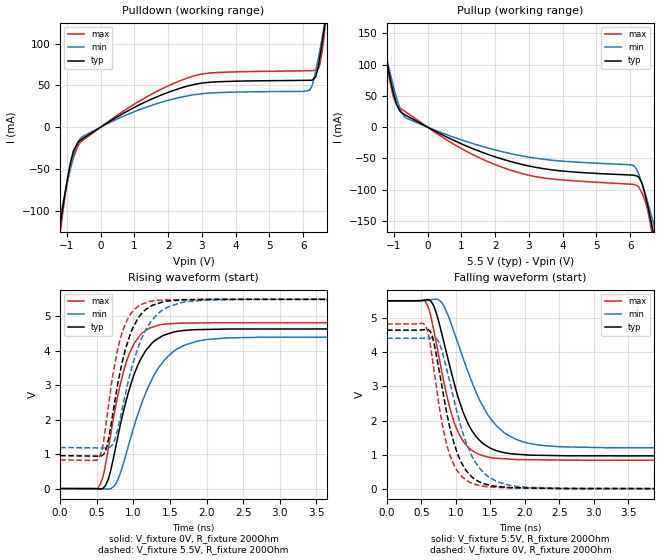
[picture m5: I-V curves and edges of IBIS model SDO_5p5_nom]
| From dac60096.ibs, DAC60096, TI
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|   Model
[Model]   SDO_5p5_nom
Model_type   Output
Polarity   Non-Inverting
Vmeas = 2.75
Vref = 0
Cref = 1pF
Rref = 100000
|   typ   min   max
C_comp   13.124pF   12.937pF   13.913pF
[Voltage Range]   5.5   5.499   5.501
[Temperature Range]   27   105   -40
[Pullup Reference]   5.5   5.499   5.501
[Pulldown Reference]   0   0   0
[Power Clamp Reference]   5.5   5.499   5.501
[GND Clamp Reference]   0   0   0
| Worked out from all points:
|   slope of the pulldown table from 0 to 0.825 V, typ, clamps not added: 41.5 ohm
|   slope of the pullup table from 0 to 0.825 V, typ, clamps not added: 36.9 ohm
|   falling waveform, V_fixture 5.5V, R_fixture 200Ohm: 20-80 % time 400ps typ, 541ps min, 325ps max; typ from 5.5 V to 0.955 V
|   rising waveform, V_fixture 0V, R_fixture 200Ohm: 20-80 % time 357ps typ, 464ps min, 292ps max; typ from 0 V to 4.64 V
|   rising waveform, V_fixture 5.5V, R_fixture 200Ohm: 20-80 % time 282ps typ, 354ps min, 233ps max; typ from 0.955 V to 5.5 V
|   falling waveform, V_fixture 0V, R_fixture 200Ohm: 20-80 % time 309ps typ, 390ps min, 263ps max; typ from 4.64 V to 0 V
[Pulldown]
|   Voltage   I(typ)   I(min)   I(max)
-5.5V     -1.396A    -1.141A    -1.674A
-1.359V   -160.1mA   -141.1mA   -181mA
-1.144V   -102mA     -96.41mA   -109.2mA
-995.5mV  -64.53mA   -67.3mA    -67.28mA
-814mV    -29.52mA   -35.59mA   -37.78mA
-566.5mV  -14.69mA   -12.25mA   -16.91mA
2.733V    50.8mA     38.61mA    61.04mA
6.182V    56.1mA     44.1mA     67.53mA
6.364V    59.98mA    65.71mA    68.08mA
6.479V    80.55mA    89.03mA    72.98mA
6.677V    133.5mA    133.4mA    129.2mA
11V       1.487A     1.216A     1.844A
[Pullup]
|   Voltage   I(typ)   I(min)   I(max)
-5.5V     1.434A     1.169A     1.793A
-1.837V   293.1mA    259.1mA    340.4mA
-1.375V   153.7mA    148mA      162.9mA
-1.095V   74.62mA    83.43mA    67.54mA
-814mV    25.31mA    29.59mA    30.55mA
-38.5mV   1.133mA    858.2uA    1.477mA
2.321V    -52.9mA    -40.63mA   -66.35mA
6.099V    -76.87mA   -61.46mA   -91.65mA
6.347V    -89.44mA   -88.99mA   -104.8mA
6.644V    -157.3mA   -144.3mA   -168.5mA
6.726V    -179.2mA   -161.1mA   -195.4mA
11V       -1.454A    -1.191A    -1.738A
[Ramp]
R_load = 200
|   typ   min   max
dV/dt_r   2.78525/3.57276e-10   2.64196/4.63284e-10   2.89374/2.91791e-10
dV/dt_f   2.72682/4e-10   2.58421/5.38847e-10   2.80226/3.25162e-10
[Falling Waveform]
V_fixture = 5.5V
V_fixture_min = 5.499V
V_fixture_max = 5.501V
R_fixture = 200Ohm
C_fixture = 0F
|   Time   V(typ)   V(min)   V(max)
0s        5.5V       5.499V     5.501V
539.6ps   5.518V     5.499V     5.5V
650.8ps   5.447V     5.53V      4.907V
810.9ps   4.406V     5.394V     3.264V
997ps     2.928V     4.444V     1.83V
1.198ns   1.826V     3.306V     1.188V
1.445ns   1.263V     2.229V     945.6mV
1.867ns   1.023V     1.459V     865.8mV
2.505ns   978.5mV    1.238V     848.7mV
10ns      955.3mV    1.192V     830.6mV
[Rising Waveform]
V_fixture = 0V
V_fixture_min = 0V
V_fixture_max = 0V
R_fixture = 200Ohm
C_fixture = 0F
|   Time   V(typ)   V(min)   V(max)
0s        -20.71nV   -110.4nV   -44.83nV
494.9ps   -5.579mV   775.8uV    -8.077mV
616.9ps   85.05mV    -11.91mV   659mV
784.3ps   1.464V     232.2mV    2.661V
939.7ps   2.841V     1.293V     3.887V
1.1ns     3.761V     2.398V     4.473V
1.339ns   4.356V     3.492V     4.743V
1.693ns   4.589V     4.158V     4.803V
2.278ns   4.631V     4.373V     4.814V
10ns      4.642V     4.403V     4.823V
[Rising Waveform]
V_fixture = 5.5V
V_fixture_min = 5.499V
V_fixture_max = 5.501V
R_fixture = 200Ohm
C_fixture = 0F
|   Time   V(typ)   V(min)   V(max)
0s        955mV      1.191V     830.5mV
511.5ps   941.3mV    1.18V      840.3mV
604.4ps   1.027V     1.178V     1.54V
745ps     2.507V     1.412V     3.612V
848.5ps   3.675V     2.316V     4.54V
994.4ps   4.673V     3.633V     5.155V
1.213ns   5.257V     4.763V     5.427V
1.472ns   5.443V     5.272V     5.48V
2.009ns   5.489V     5.474V     5.493V
10ns      5.5V       5.499V     5.501V
[Falling Waveform]
|Gnd
V_fixture = 0V
V_fixture_min = 0V
V_fixture_max = 0V
R_fixture = 200Ohm
C_fixture = 0F
|   Time   V(typ)   V(min)   V(max)
0s        4.642V     4.404V     4.823V
517.3ps   4.651V     4.403V     4.839V
627.7ps   4.599V     4.415V     4.213V
755.8ps   3.47V      4.275V     2.443V
909.4ps   1.819V     3.143V     1.012V
1.081ns   764.6mV    1.764V     376.9mV
1.339ns   215.7mV    622.4mV    107.3mV
1.591ns   78.7mV     225.1mV    54.1mV
2.09ns    33.36mV    47.77mV    29.01mV
10ns      471.5uV    1.351mV    100.8uV
